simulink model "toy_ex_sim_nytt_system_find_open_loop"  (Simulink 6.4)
settings: Solver=ode45  StartTime=0.0  StopTime=10.0  RelTol=1e-3
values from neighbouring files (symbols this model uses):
  alpha = -0.9    [bounds.m]    (also in real_ex_linkomb_W_and_DP.m = 1; real_ex_linkomb_W_and_RHOT.m = -0.2; real_ex_without_noise_z_30.m = -6:0.01:4; toy_ex_nytt_system.m)
  den_G1 = [-1 1]    [bounds.m]    (also in toy_ex_nytt_system.m; toy_ex_nytt_system_without_noise.m; toy_ex_nytt_system_with_disturbance.m; toy_ex_nytt_system_with_measure_noise.m)
  den_G2 = [-1 1]    [bounds.m]    (also in toy_ex_nytt_system.m; toy_ex_nytt_system_without_noise.m; toy_ex_nytt_system_with_disturbance.m; toy_ex_nytt_system_with_measure_noise.m)
  K_indre = 10    [real_ex_linkomb_W_and_DP.m]    (also in real_ex_linkomb_W_and_RHOT.m = 5; toy_ex_nytt_system.m = 50; toy_ex_nytt_system_without_noise.m = 20; toy_ex_nytt_system_with_disturbance.m = 50)
  K_ytre = 0.01    [real_ex_linkomb_W_and_DP.m]    (also in real_ex_linkomb_W_and_RHOT.m; toy_ex_nytt_system.m = 0.1; toy_ex_nytt_system_without_noise.m = 0.1; toy_ex_nytt_system_with_disturbance.m = 0.1)
  num_G1 = 5*[-1.5 1]    [bounds.m]    (also in toy_ex_nytt_system.m; toy_ex_nytt_system_without_noise.m; toy_ex_nytt_system_with_disturbance.m; toy_ex_nytt_system_with_measure_noise.m)
  num_G2 = 5*[-0.5 1]    [bounds.m]    (also in toy_ex_nytt_system.m; toy_ex_nytt_system_without_noise.m; toy_ex_nytt_system_with_disturbance.m; toy_ex_nytt_system_with_measure_noise.m)
  Ti = 100    [real_ex_linkomb_W_and_DP.m]    (also in real_ex_linkomb_W_and_RHOT.m = 100000; toy_ex_nytt_system.m = 10; toy_ex_nytt_system_without_noise.m = 10; toy_ex_nytt_system_with_disturbance.m = 10)

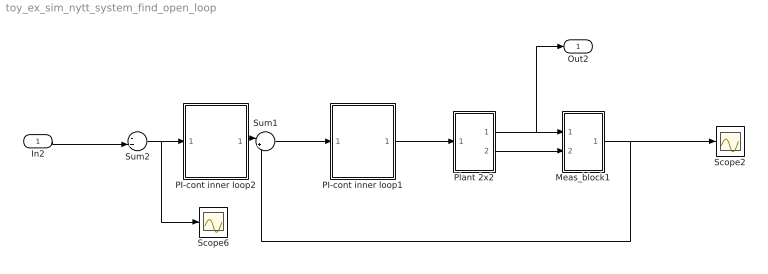
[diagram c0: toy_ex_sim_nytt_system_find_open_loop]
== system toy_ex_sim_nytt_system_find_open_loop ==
  In2 : Inport
  Meas_block1 : Subsystem
  PI-cont inner loop1 : Subsystem
  PI-cont inner loop2 : Subsystem
  Plant 2x2 : Subsystem
  Scope2 : Scope
  Scope6 : Scope
  Sum1 : Sum  Inputs=|+-
  Sum2 : Sum  Inputs=-+|
  Out2 : Outport
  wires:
  Plant 2x2/2(y2) -> Meas_block1/2(In2)
  Plant 2x2/1("y1 ") -> Meas_block1/1(In1), Out2/1
  Meas_block1/1(Out1) -> Scope2/1, Sum1/2
  Sum1/1 -> PI-cont inner loop1/1(In1)
  PI-cont inner loop1/1(Out1) -> Plant 2x2/1(In1)
  PI-cont inner loop2/1(Out1) -> Sum1/1
  Sum2/1 -> PI-cont inner loop2/1(In1), Scope6/1
  In2/1 -> Sum2/2

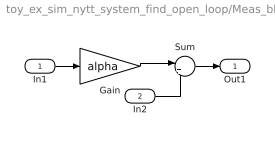
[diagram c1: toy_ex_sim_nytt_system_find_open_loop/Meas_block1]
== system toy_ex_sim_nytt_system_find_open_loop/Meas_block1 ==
  In1 : Inport
  In2 : Inport  Port=2
  Gain : Gain  Gain=alpha
  Sum : Sum  Inputs=|++
  Out1 : Outport
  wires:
  In2/1 -> Sum/2
  Sum/1 -> Out1/1
  In1/1 -> Gain/1
  Gain/1 -> Sum/1

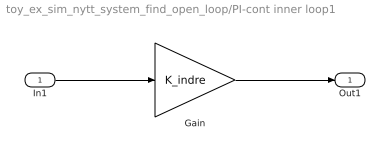
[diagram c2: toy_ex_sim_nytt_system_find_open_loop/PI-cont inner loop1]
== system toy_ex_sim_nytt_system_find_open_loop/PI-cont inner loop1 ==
  In1 : Inport
  Gain : Gain  Gain=K_indre
  Out1 : Outport
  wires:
  In1/1 -> Gain/1
  Gain/1 -> Out1/1

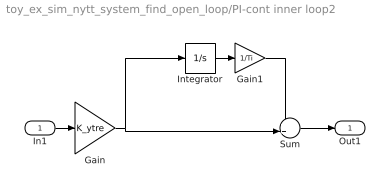
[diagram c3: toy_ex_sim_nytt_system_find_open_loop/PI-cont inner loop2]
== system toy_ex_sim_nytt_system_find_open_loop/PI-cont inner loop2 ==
  In1 : Inport
  Gain : Gain  Gain=K_ytre
  Gain1 : Gain  Gain=1/Ti
  Integrator : Integrator
  Sum : Sum  Inputs=++|
  Out1 : Outport
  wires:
  Gain/1 -> Integrator/1, Sum/2
  In1/1 -> Gain/1
  Integrator/1 -> Gain1/1
  Gain1/1 -> Sum/1
  Sum/1 -> Out1/1

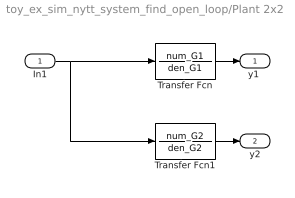
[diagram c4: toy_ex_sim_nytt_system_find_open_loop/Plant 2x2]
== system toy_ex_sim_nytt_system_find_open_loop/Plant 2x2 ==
  In1 : Inport
  Transfer Fcn : TransferFcn  Numerator=num_G1  Denominator=den_G1
  Transfer Fcn1 : TransferFcn  Numerator=num_G2  Denominator=den_G2
  "y1 " : Outport
  y2 : Outport  Port=2
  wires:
  Transfer Fcn1/1 -> y2/1
  Transfer Fcn/1 -> "y1 "/1
  In1/1 -> Transfer Fcn/1, Transfer Fcn1/1
